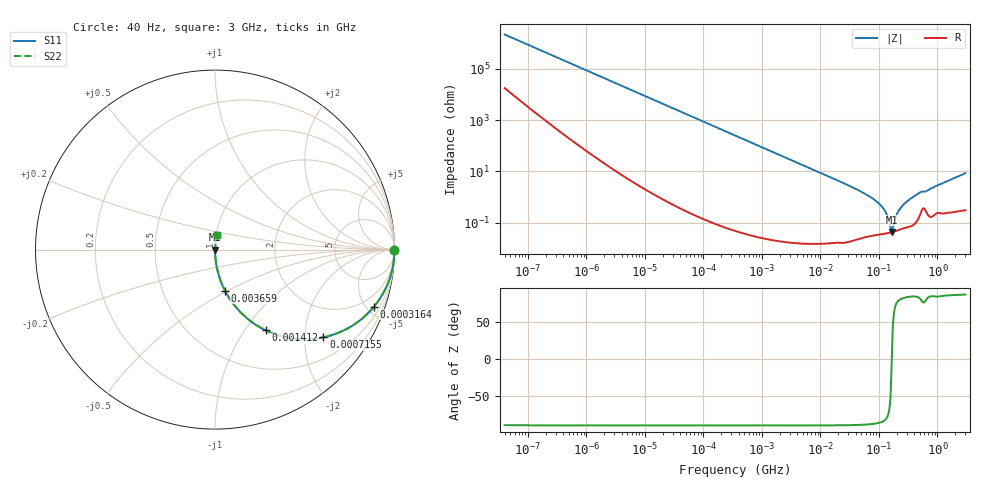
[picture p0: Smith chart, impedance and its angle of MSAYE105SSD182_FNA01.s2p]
! MSAYE105SSD182_FNA01  S-PARAMETER MODEL  ( General Type )
! Model Generated by TAIYO YUDEN Corporation (http://www.ty-top.com)
! Version 2.0
! TAIYO YUDEN Control No. 040624
! Copyright(c) 2004 TAIYO YUDEN CO.,LTD. All Rights Reserved.
! Product Description (link to TY-COMPAS)
! https://ds.yuden.co.jp/TYCOMPAS/or/detail?pn=MSAYE105SSD182KFNA01&u=M
! Products Name : Multilayer Ceramic Capacitors
! Characteristics :
!  Capacitance : 1800 pF , Rated Voltage : 16V
!  Case Size : 1.0 x 0.5 / 0.039 x 0.02 [mm/inch] , Thickness : 0.5 / 0.02 [mm/inch]
!  (Conditions: Temperature = 25 degC , DC Bias Current/Voltage = 0A / 0V)
! External Node Assignments :
!  1  o---| |---o  2
! GND o---------o GND
! Frequency Range : 40Hz  -  3GHz  [ 401 STEP ]
# MHz S RI R 50
! Freq[MHz].  S11 Real  S11 Imag  S21 Real  S21 Imag  S12 Real  S12 Imag  S22 Real  S22 Imag
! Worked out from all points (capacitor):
!   401 points, 40 Hz to 3 GHz, reference 50 ohm
!   read as one part in series: C = 1.8 nF near 44 Hz
!   lowest |Z| = 42.7 mohm at 164.9 MHz (marker M1)
!   series resonance near 165.6 MHz, so ESL is about 510 pH
!   S11 on the Smith chart (normalised r, x): 40 Hz: open; 316.4 kHz: 1.00, -5.59; 715.5 kHz: 1.00, -2.47; 1.412 MHz: 1.00, -1.25; 3.659 MHz: 1.00, -0.48; 3 GHz: 1.01, +0.17
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4e-05  1 -4.53e-05  3.67e-07 4.53e-05  3.67e-07 4.53e-05  1 -4.53e-05
9.5e-05  1 -0.000108  4.34e-07 0.000108  4.34e-07 0.000108  1 -0.000108
0.000834  1 -0.000944  1.63e-06 0.000944  1.63e-06 0.000944  1 -0.000944
0.017386  0.9996 -0.0197  0.000391 0.0197  0.000391 0.0197  0.9996 -0.0197
0.093035  0.989 -0.1041  0.011 0.1041  0.011 0.1041  0.989 -0.1041
0.316385  0.8863 -0.3173  0.1137 0.3173  0.1137 0.3173  0.8863 -0.3173
0.362475  0.8559 -0.3511  0.1441 0.3511  0.1441 0.3511  0.8559 -0.3511
0.715473  0.604 -0.4889  0.396 0.4889  0.396 0.4889  0.604 -0.4889
1.412238  0.2814 -0.4495  0.7186 0.4495  0.7186 0.4495  0.2814 -0.4495
3.658884  0.0552 -0.228  0.9448 0.228  0.9448 0.228  0.0552 -0.228
7.222098  0.0148 -0.1203  0.9852 0.1203  0.9852 0.1203  0.0148 -0.1203
76.28187  0.000388 -0.00905  0.9996 0.00905  0.9996 0.00905  0.000388 -0.00905
120.0322  0.000374 -0.00343  0.9996 0.00343  0.9996 0.00343  0.000374 -0.00343
137.5184  0.000386 -0.00195  0.9996 0.00195  0.9996 0.00195  0.000386 -0.00195
150.5692  0.0004 -0.00099  0.9996 0.00099  0.9996 0.00099  0.0004 -0.00099
164.8585  0.000424 -4.85e-05  0.9996 4.85e-05  0.9996 4.85e-05  0.000424 -4.85e-05
180.504  0.000452 0.000908  0.9995 -0.000908  0.9995 -0.000908  0.000452 0.000908
197.6342  0.000483 0.00187  0.9995 -0.00187  0.9995 -0.00187  0.000483 0.00187
226.4253  0.000539 0.00332  0.9995 -0.00332  0.9995 -0.00332  0.000539 0.00332
356.2883  0.000807 0.00894  0.9992 -0.00894  0.9992 -0.00894  0.000807 0.00894
512.0387  0.00242 0.0152  0.9976 -0.0152  0.9976 -0.0152  0.00242 0.0152
3000  0.0101 0.084  0.9899 -0.084  0.9899 -0.084  0.0101 0.084
